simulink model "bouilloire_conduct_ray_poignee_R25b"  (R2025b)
settings: Solver=VariableStepAuto  StartTime=0.0  StopTime=2000  RelTol=1e-3  AbsTol=1e-3  EnableMultiTasking=on
PreLoadFcn:
  | % Caractéristiques de la poignée en polypropylène
  | D= 0.027;         % [m]  Diamètre moyen
  | L1= 0.03;         % [m]  Longueur des tronçons d'extrémité
  | L2= 0.11;         % [m]  Longueur du tronçon central
  | A= pi*D^2/4;      % [m^2] Surface de la section
  | A_cyl1= pi*D*L1;  % [m^2] Surface cylindre des tronçons d'extrémité
  | A_cyl2= pi*D*L2;  % [m^2] Surface cylindre du tronçon central
  | k= 0.2;           % [W/(K*m)] Conductivité thermique
  | m1= 900*A*L1;     % [kg] Masse tronçons d'extrémité (Masse vol = 900 kg/m3)
  | m2= 900*A*L2;     % [kg] Masse tronçon central
  | c= 1700;          % [J/kg/K] Chaleur spécifique
  | h= 6.8;           % [W/(m^2/K)] Coefficient de convection thermique
  | T_air= 20;        % [degC]
  | T_base= 80;       % [degC]
  | T_init= 20;       % [degC]
  | % Point de fusion du polypropylène = 160 degC
  | e= 0.94;          % Emissivité du plastique noir
libraries: fl_lib x31, nesl_utility x7

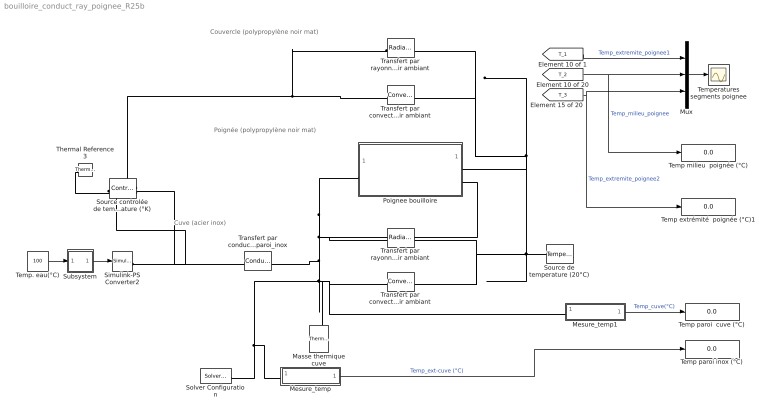
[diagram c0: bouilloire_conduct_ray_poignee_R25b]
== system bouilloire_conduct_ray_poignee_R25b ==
  note: Poignée (polypropylène noir mat)
  note: Cuve (acier inox)
  note: Couvercle (polypropylène noir mat)
  Masse thermique cuve : fl_lib/Thermal/Thermal Elements/Thermal Mass  mass_type=foundation.enum.constant_variable.constant  mass=0.17 kg  sp_heat=470 J/kg/K  mass_min=1e-6 kg  num_ports=foundation.enum.numPorts2.one  m_specify=off  m_priority=High  m=1 kg  m_nominal_specify=off  m_nominal_value=1  m_nominal_unit=kg  T_specify=on  T_priority=High  T=293 K  T_nominal_specify=off  T_nominal_value=1  T_nominal_unit=K  Q_specify=on  Q_priority=None  Q=0 W  Q_nominal_specify=off  Q_nominal_value=1  Q_nominal_unit=W
  Mesure_temp : Subsystem
  Mesure_temp1 : Subsystem
  Mux : Mux  Inputs=3
  Poignee bouilloire : Subsystem  Tag=PublishSubsystem
  Simulink-PS Converter2 : nesl_utility/Simulink-PS Converter  PhysicalDomain=network_engine_domain  SubClassName=ps_input  LeftPortType=input  RightPortType=output  PseudoPeriodic=off  Frequencies=[]  NoiseDistribution=none  NoiseParameters=[]  Unit=1  AffineConversion=off  FilteringAndDerivatives=zero  SimscapeFilterOrder=1  InputFilterTimeConstant=0.001  UdotUserProvided=1
  Solver Configuration : nesl_utility/Solver Configuration  PhysicalDomain=network_engine_domain  SubClassName=solver  LeftPortType=input  RightPortType=generic  Tones=[]  Harmonics=[]  SimulateNoise=off  Profile=off  UseLocalSampling=off  EnableSwitchedLinearOptims=on  FrequencyDomain=off  UseCCode=off  RelTol=0.001  AbsTol=1e-06  MinStep=1e-09  ToWorkspace=off  RevertToSquareIcSolve=off  NumHomotopyIterations=100  PhasorMode=off  PhasorModeNumHarmonics=1  ConsistencySolver=NEWTON_FTOL  IndexReductionMethod=DerivativeReplacement  DoDC=off  ResidualTolerance=1e-09  ConsistencyTolSource=GLOBAL  ConsistencyAbsTol=0.001  ConsistencyRelTol=0.001  ConsistencyTolFactor=0.001  UseLocalSolver=off  LocalSolverChoice=NE_BACKWARD_EULER_ADVANCER  ResolveIndetEquations=on  FunctionEvalNumThread=1  LocalSolverSampleTime=0.001  DoFixedCost=off  MaxNonlinIter=3  MaxModeIter=2  ComputeImpulses=off  ImpulseIterations=2  LinearAlgebra=Sparse  LinearAlgebraNumThread=0  EquationFormulation=NE_TIME_EF  DelaysMemoryBudget=1024  AutomaticFiltering=on  FilteringTimeConstant=0.001  PartitionStorageMethod=AS_NEEDED  PartitionMemoryBudget=1024  PartitionMethod=FAST  MultibodyUseLocalSolver=off  MultibodyLocalSolverChoice=ODE1  MultibodyLocalSolverSampleTime=0.001
  Source controlée de temperature (°K) : fl_lib/Thermal/Thermal Sources/Controlled Temperature Source
  Source de temperature (20°C) : fl_lib/Thermal/Thermal Sources/Temperature Source  temperature=293.15 K
  Subsystem : Subsystem
  Temp extrémité  poignée (°C)1 : Display
  Temp milieu  poignée (°C) : Display
  Temp paroi  cuve (°C) : Display
  Temp paroi inox (°C) : Display
  Temp. eau(°C) : Constant  Value=100
  Temperatures segments poignee : Scope
  Thermal Reference3 : fl_lib/Thermal/Thermal Elements/Thermal Reference
  Transfert par conduction eau-paroi_inox : fl_lib/Thermal/Thermal Elements/Conductive Heat Transfer  thermal_type=foundation.enum.ConstantVariableTabulated.Constant  wall_geometry=foundation.enum.ConductionWallGeometry.Planar  area=53e-3 m^2  thickness=0.4 mm  d_in=0.05 m  d_out=0.1 m  L=1 m  th_cond_min=10 W/(K*m)  th_cond=17 W/(m*K)  th_cond_TLU=[413, 401, 392, 383, 371, 357, 342] W/(K*m)  temp_TLU=[200, 273, 400, 600, 800, 1000, 1200] K  T_specify=off  T_priority=None  T=0 K  T_nominal_specify=off  T_nominal_value=1  T_nominal_unit=K  Q_specify=off  Q_priority=None  Q=0 W  Q_nominal_specify=off  Q_nominal_value=1  Q_nominal_unit=W
  Transfert par convection couvercle-air ambiant : fl_lib/Thermal/Thermal Elements/Convective Heat Transfer  thermal_type=foundation.enum.constant_variable.constant  area=8e-3 m^2  heat_tr_coeff=6.8 W/(m^2 * K)  min_heat_tr_coeff=1e-3 W/(K*m^2)  T_specify=off  T_priority=None  T=0 K  T_nominal_specify=off  T_nominal_value=1  T_nominal_unit=K  Q_specify=off  Q_priority=None  Q=0 W  Q_nominal_specify=off  Q_nominal_value=1  Q_nominal_unit=W
  Transfert par convection paroi_inox-air ambiant : fl_lib/Thermal/Thermal Elements/Convective Heat Transfer  thermal_type=foundation.enum.constant_variable.constant  area=53e-3 m^2  heat_tr_coeff=6.8 W/(m^2 * K)  min_heat_tr_coeff=1e-3 W/(K*m^2)  T_specify=off  T_priority=None  T=0 K  T_nominal_specify=off  T_nominal_value=1  T_nominal_unit=K  Q_specify=off  Q_priority=None  Q=0 W  Q_nominal_specify=off  Q_nominal_value=1  Q_nominal_unit=W
  Transfert par rayonnement couvercle-air ambiant : fl_lib/Thermal/Thermal Elements/Radiative Heat Transfer  area=8e-3 m^2  rad_tr_coeff=e*5.67e-8 W/(m^2*K^4)  T_specify=off  T_priority=None  T=0 K  T_nominal_specify=off  T_nominal_value=1  T_nominal_unit=K  Q_specify=off  Q_priority=None  Q=0 W  Q_nominal_specify=off  Q_nominal_value=1  Q_nominal_unit=W
  Transfert par rayonnement paroi_inox-air ambiant : fl_lib/Thermal/Thermal Elements/Radiative Heat Transfer  area=53e-3 m^2  rad_tr_coeff=0.87*5.67e-8 W/(m^2*K^4)  T_specify=off  T_priority=None  T=0 K  T_nominal_specify=off  T_nominal_value=1  T_nominal_unit=K  Q_specify=off  Q_priority=None  Q=0 W  Q_nominal_specify=off  Q_nominal_value=1  Q_nominal_unit=W
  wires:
  Mesure_temp/1(Temp(°C)) -> Temp paroi inox (°C)/1  "Temp_ext-cuve (°C)"
  Mesure_temp1/1(Temp(°C)) -> Temp paroi  cuve (°C)/1  "Temp_cuve(°C)"
  Subsystem/1(S1) -> Simulink-PS Converter2/1
  Temp. eau(°C)/1 -> Subsystem/1(E1)
  [T_2] -> Mux/2, Temp milieu  poignée (°C)/1  "Temp_milieu_poignee"
  [T_3] -> Mux/3, Temp extrémité  poignée (°C)1/1  "Temp_extremite_poignee2"
  [T_1] -> Mux/1  "Temp_extremite_poignee1"
  Mux/1 -> Temperatures segments poignee/1
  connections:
  Poignee bouilloire/LConn1 -- Poignee bouilloire/RConn2 -- Transfert par rayonnement paroi_inox-air ambiant/LConn1 -- Transfert par conduction eau-paroi_inox/RConn1 -- Mesure_temp/LConn1 -- Solver Configuration/RConn1 -- Mesure_temp1/LConn1 -- Masse thermique cuve/LConn1 -- Transfert par convection paroi_inox-air ambiant/LConn1
  Transfert par convection couvercle-air ambiant/RConn1 -- Transfert par rayonnement couvercle-air ambiant/RConn1 -- Source de temperature (20°C)/LConn1 -- Transfert par convection paroi_inox-air ambiant/RConn1 -- Transfert par rayonnement paroi_inox-air ambiant/RConn1 -- Poignee bouilloire/RConn1
  Thermal Reference3/LConn1 -- Source controlée de temperature (°K)/RConn2
  Source controlée de temperature (°K)/RConn1 -- Simulink-PS Converter2/RConn1
  Source controlée de temperature (°K)/LConn1 -- Transfert par conduction eau-paroi_inox/LConn1 -- Transfert par convection couvercle-air ambiant/LConn1 -- Transfert par rayonnement couvercle-air ambiant/LConn1

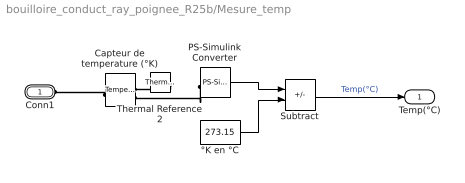
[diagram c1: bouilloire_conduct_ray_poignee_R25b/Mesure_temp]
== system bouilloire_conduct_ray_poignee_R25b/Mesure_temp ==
  Capteur de temperature (°K) : fl_lib/Thermal/Thermal Sensors/Temperature Sensor  temperature_measure=foundation.enum.MeasurementReference.difference
  PS-Simulink Converter : nesl_utility/PS-Simulink Converter  PhysicalDomain=network_engine_domain  SubClassName=ps_output  LeftPortType=input  RightPortType=output  PseudoPeriodic=off  Frequencies=[]  VectorFormat=1-D array  Unit=1  AffineConversion=off
  Subtract : Sum  Inputs=+-
  Thermal Reference2 : fl_lib/Thermal/Thermal Elements/Thermal Reference
  °K en °C : Constant  Value=273.15
  Conn1 : PMIOPort  Side=Left
  Temp(°C) : Outport  VectorParamsAs1DForOutWhenUnconnected=off
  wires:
  °K en °C/1 -> Subtract/2
  Subtract/1 -> Temp(°C)/1  "Temp(°C)"
  PS-Simulink Converter/1 -> Subtract/1
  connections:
  PS-Simulink Converter/LConn1 -- Capteur de temperature (°K)/RConn2
  Thermal Reference2/LConn1 -- Capteur de temperature (°K)/RConn1
  Capteur de temperature (°K)/LConn1 -- Conn1/RConn1

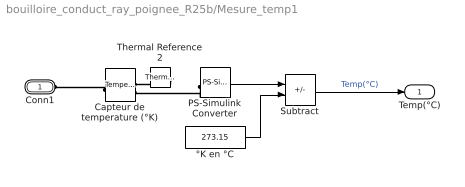
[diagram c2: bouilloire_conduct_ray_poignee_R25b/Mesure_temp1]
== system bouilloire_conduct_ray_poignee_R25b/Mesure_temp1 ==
  Capteur de temperature (°K) : fl_lib/Thermal/Thermal Sensors/Temperature Sensor  temperature_measure=foundation.enum.MeasurementReference.difference
  PS-Simulink Converter : nesl_utility/PS-Simulink Converter  PhysicalDomain=network_engine_domain  SubClassName=ps_output  LeftPortType=input  RightPortType=output  PseudoPeriodic=off  Frequencies=[]  VectorFormat=1-D array  Unit=1  AffineConversion=off
  Subtract : Sum  Inputs=+-
  Thermal Reference2 : fl_lib/Thermal/Thermal Elements/Thermal Reference
  °K en °C : Constant  Value=273.15
  Conn1 : PMIOPort  Side=Left
  Temp(°C) : Outport  VectorParamsAs1DForOutWhenUnconnected=off
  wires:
  °K en °C/1 -> Subtract/2
  Subtract/1 -> Temp(°C)/1  "Temp(°C)"
  PS-Simulink Converter/1 -> Subtract/1
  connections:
  PS-Simulink Converter/LConn1 -- Capteur de temperature (°K)/RConn2
  Thermal Reference2/LConn1 -- Capteur de temperature (°K)/RConn1
  Capteur de temperature (°K)/LConn1 -- Conn1/RConn1

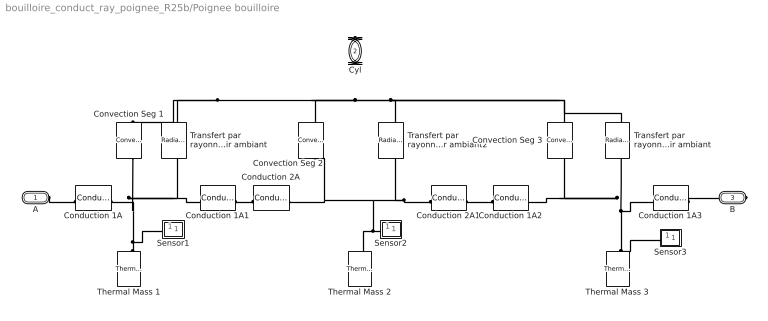
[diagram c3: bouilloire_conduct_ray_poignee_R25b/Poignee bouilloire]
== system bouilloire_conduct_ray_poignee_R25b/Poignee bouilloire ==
  Conduction 1A{,1..3} (4 alike) : fl_lib/Thermal/Thermal Elements/Conductive Heat Transfer  thermal_type=foundation.enum.ConstantVariableTabulated.Constant  wall_geometry=foundation.enum.ConductionWallGeometry.Planar  area=A m^2  thickness=L1/2 m  d_in=0.05 m  d_out=0.1 m  L=1 m  th_cond_min=10 W/(K*m)  th_cond=k W/m/K  th_cond_TLU=[413, 401, 392, 383, 371, 357, 342] W/(K*m)  temp_TLU=[200, 273, 400, 600, 800, 1000, 1200] K  T_specify=off  T_priority=High  T=0 K  T_nominal_specify=off  T_nominal_value=1  T_nominal_unit=K  Q_specify=off  Q_priority=High  Q=0 J/s  Q_nominal_specify=off  Q_nominal_value=1  Q_nominal_unit=J/s
  Conduction 2A : fl_lib/Thermal/Thermal Elements/Conductive Heat Transfer  thermal_type=foundation.enum.ConstantVariableTabulated.Constant  wall_geometry=foundation.enum.ConductionWallGeometry.Planar  area=A m^2  thickness=L2/2 m  d_in=0.05 m  d_out=0.1 m  L=1 m  th_cond_min=10 W/(K*m)  th_cond=k W/m/K  th_cond_TLU=[413, 401, 392, 383, 371, 357, 342] W/(K*m)  temp_TLU=[200, 273, 400, 600, 800, 1000, 1200] K  T_specify=off  T_priority=High  T=0 K  T_nominal_specify=off  T_nominal_value=1  T_nominal_unit=K  Q_specify=off  Q_priority=High  Q=0 J/s  Q_nominal_specify=off  Q_nominal_value=1  Q_nominal_unit=J/s
  Conduction 2A1 : fl_lib/Thermal/Thermal Elements/Conductive Heat Transfer  thermal_type=foundation.enum.ConstantVariableTabulated.Constant  wall_geometry=foundation.enum.ConductionWallGeometry.Planar  area=A m^2  thickness=L2/2 m  d_in=0.05 m  d_out=0.1 m  L=1 m  th_cond_min=10 W/(K*m)  th_cond=k W/m/K  th_cond_TLU=[413, 401, 392, 383, 371, 357, 342] W/(K*m)  temp_TLU=[200, 273, 400, 600, 800, 1000, 1200] K  T_specify=off  T_priority=High  T=0 K  T_nominal_specify=off  T_nominal_value=1  T_nominal_unit=K  Q_specify=off  Q_priority=High  Q=0 J/s  Q_nominal_specify=off  Q_nominal_value=1  Q_nominal_unit=J/s
  Convection Seg 1 : fl_lib/Thermal/Thermal Elements/Convective Heat Transfer  thermal_type=foundation.enum.constant_variable.constant  area=A_cyl1 m^2  heat_tr_coeff=h W/m^2/K  min_heat_tr_coeff=1e-3 W/(K*m^2)  T_specify=off  T_priority=High  T=0 K  T_nominal_specify=off  T_nominal_value=1  T_nominal_unit=K  Q_specify=off  Q_priority=High  Q=0 J/s  Q_nominal_specify=off  Q_nominal_value=1  Q_nominal_unit=J/s
  Convection Seg 2 : fl_lib/Thermal/Thermal Elements/Convective Heat Transfer  thermal_type=foundation.enum.constant_variable.constant  area=A_cyl2 m^2  heat_tr_coeff=h W/m^2/K  min_heat_tr_coeff=1e-3 W/(K*m^2)  T_specify=off  T_priority=High  T=0 K  T_nominal_specify=off  T_nominal_value=1  T_nominal_unit=K  Q_specify=off  Q_priority=High  Q=0 J/s  Q_nominal_specify=off  Q_nominal_value=1  Q_nominal_unit=J/s
  Convection Seg 3 : fl_lib/Thermal/Thermal Elements/Convective Heat Transfer  thermal_type=foundation.enum.constant_variable.constant  area=A_cyl1 m^2  heat_tr_coeff=h W/m^2/K  min_heat_tr_coeff=1e-3 W/(K*m^2)  T_specify=off  T_priority=High  T=0 K  T_nominal_specify=off  T_nominal_value=1  T_nominal_unit=K  Q_specify=off  Q_priority=High  Q=0 J/s  Q_nominal_specify=off  Q_nominal_value=1  Q_nominal_unit=J/s
  Sensor1 : Subsystem
  Sensor2 : Subsystem
  Sensor3 : Subsystem
  Thermal Mass 1 : fl_lib/Thermal/Thermal Elements/Thermal Mass  mass_type=foundation.enum.constant_variable.constant  mass=m1 kg  sp_heat=c J/kg/K  mass_min=1e-6 kg  num_ports=foundation.enum.numPorts2.one  m_specify=off  m_priority=High  m=1 kg  m_nominal_specify=off  m_nominal_value=1  m_nominal_unit=kg  T_specify=on  T_priority=High  T=T_init degC  T_nominal_specify=off  T_nominal_value=1  T_nominal_unit=K  Q_specify=off  Q_priority=None  Q=0 W  Q_nominal_specify=off  Q_nominal_value=1  Q_nominal_unit=W
  Thermal Mass 2 : fl_lib/Thermal/Thermal Elements/Thermal Mass  mass_type=foundation.enum.constant_variable.constant  mass=m2 kg  sp_heat=c J/kg/K  mass_min=1e-6 kg  num_ports=foundation.enum.numPorts2.one  m_specify=off  m_priority=High  m=1 kg  m_nominal_specify=off  m_nominal_value=1  m_nominal_unit=kg  T_specify=on  T_priority=High  T=T_init degC  T_nominal_specify=off  T_nominal_value=1  T_nominal_unit=K  Q_specify=off  Q_priority=None  Q=0 W  Q_nominal_specify=off  Q_nominal_value=1  Q_nominal_unit=W
  Thermal Mass 3 : fl_lib/Thermal/Thermal Elements/Thermal Mass  mass_type=foundation.enum.constant_variable.constant  mass=m1 kg  sp_heat=c J/kg/K  mass_min=1e-6 kg  num_ports=foundation.enum.numPorts2.one  m_specify=off  m_priority=High  m=1 kg  m_nominal_specify=off  m_nominal_value=1  m_nominal_unit=kg  T_specify=on  T_priority=High  T=T_init degC  T_nominal_specify=off  T_nominal_value=1  T_nominal_unit=K  Q_specify=off  Q_priority=None  Q=0 W  Q_nominal_specify=off  Q_nominal_value=1  Q_nominal_unit=W
  Transfert par rayonnement seg1-air ambiant : fl_lib/Thermal/Thermal Elements/Radiative Heat Transfer  area=A_cyl1 m^2  rad_tr_coeff=e*5.67e-8 W/(m^2*K^4)  T_specify=off  T_priority=None  T=0 K  T_nominal_specify=off  T_nominal_value=1  T_nominal_unit=K  Q_specify=off  Q_priority=None  Q=0 W  Q_nominal_specify=off  Q_nominal_value=1  Q_nominal_unit=W
  Transfert par rayonnement seg2-air ambiant2 : fl_lib/Thermal/Thermal Elements/Radiative Heat Transfer  area=A_cyl2 m^2  rad_tr_coeff=e*5.67e-8 W/(m^2*K^4)  T_specify=off  T_priority=None  T=0 K  T_nominal_specify=off  T_nominal_value=1  T_nominal_unit=K  Q_specify=off  Q_priority=None  Q=0 W  Q_nominal_specify=off  Q_nominal_value=1  Q_nominal_unit=W
  Transfert par rayonnement seg3-air ambiant : fl_lib/Thermal/Thermal Elements/Radiative Heat Transfer  area=A_cyl1 m^2  rad_tr_coeff=e*5.67e-8 W/(m^2*K^4)  T_specify=off  T_priority=None  T=0 K  T_nominal_specify=off  T_nominal_value=1  T_nominal_unit=K  Q_specify=off  Q_priority=None  Q=0 W  Q_nominal_specify=off  Q_nominal_value=1  Q_nominal_unit=W
  A : PMIOPort  Side=Left
  Cyl : PMIOPort  Port=2  Side=Right
  B : PMIOPort  Port=3  Side=Right
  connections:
  Conduction 2A1/RConn1 -- Conduction 1A2/LConn1
  A/RConn1 -- Conduction 1A/LConn1
  Conduction 2A/LConn1 -- Conduction 1A1/RConn1
  Thermal Mass 3/LConn1 -- Transfert par rayonnement seg3-air ambiant/LConn1 -- Convection Seg 3/LConn1 -- Conduction 1A2/RConn1 -- Conduction 1A3/LConn1 -- Sensor3/LConn1
  Sensor2/LConn1 -- Thermal Mass 2/LConn1 -- Conduction 2A/RConn1 -- Convection Seg 2/LConn1 -- Conduction 2A1/LConn1 -- Transfert par rayonnement seg2-air ambiant2/LConn1
  Thermal Mass 1/LConn1 -- Sensor1/LConn1 -- Transfert par rayonnement seg1-air ambiant/LConn1 -- Conduction 1A1/LConn1 -- Conduction 1A/RConn1 -- Convection Seg 1/LConn1
  Conduction 1A3/RConn1 -- B/RConn1
  Cyl/RConn1 -- Convection Seg 2/RConn1 -- Transfert par rayonnement seg1-air ambiant/RConn1 -- Convection Seg 1/RConn1 -- Transfert par rayonnement seg3-air ambiant/RConn1 -- Convection Seg 3/RConn1 -- Transfert par rayonnement seg2-air ambiant2/RConn1

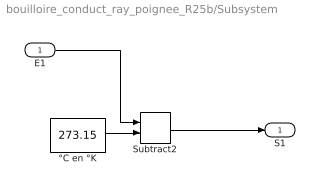
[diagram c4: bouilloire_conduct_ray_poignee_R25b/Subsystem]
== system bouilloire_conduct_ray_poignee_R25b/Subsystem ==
  E1 : Inport
  Subtract2 : Sum
  °C en °K : Constant  Value=273.15
  S1 : Outport  VectorParamsAs1DForOutWhenUnconnected=off
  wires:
  °C en °K/1 -> Subtract2/2
  Subtract2/1 -> S1/1
  E1/1 -> Subtract2/1

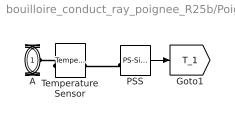
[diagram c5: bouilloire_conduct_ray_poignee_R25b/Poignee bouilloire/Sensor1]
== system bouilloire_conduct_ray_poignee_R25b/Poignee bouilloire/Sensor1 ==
  PSS : nesl_utility/PS-Simulink Converter  PhysicalDomain=network_engine_domain  SubClassName=ps_output  LeftPortType=input  RightPortType=output  PseudoPeriodic=off  Frequencies=[]  VectorFormat=1-D array  Unit=degC  AffineConversion=on
  Temperature Sensor : fl_lib/Thermal/Thermal Sensors/Temperature Sensor  temperature_measure=foundation.enum.MeasurementReference.absolute
  A : PMIOPort  Side=Left
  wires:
  PSS/1 -> [T_1]
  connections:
  PSS/LConn1 -- Temperature Sensor/RConn1
  Temperature Sensor/LConn1 -- A/RConn1

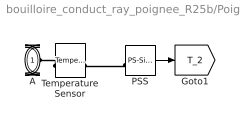
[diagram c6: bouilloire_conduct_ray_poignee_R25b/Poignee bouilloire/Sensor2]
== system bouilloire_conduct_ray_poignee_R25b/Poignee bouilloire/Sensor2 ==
  PSS : nesl_utility/PS-Simulink Converter  PhysicalDomain=network_engine_domain  SubClassName=ps_output  LeftPortType=input  RightPortType=output  PseudoPeriodic=off  Frequencies=[]  VectorFormat=1-D array  Unit=degC  AffineConversion=on
  Temperature Sensor : fl_lib/Thermal/Thermal Sensors/Temperature Sensor  temperature_measure=foundation.enum.MeasurementReference.absolute
  A : PMIOPort  Side=Left
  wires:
  PSS/1 -> [T_2]
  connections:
  PSS/LConn1 -- Temperature Sensor/RConn1
  Temperature Sensor/LConn1 -- A/RConn1

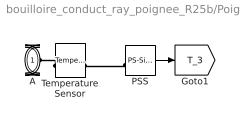
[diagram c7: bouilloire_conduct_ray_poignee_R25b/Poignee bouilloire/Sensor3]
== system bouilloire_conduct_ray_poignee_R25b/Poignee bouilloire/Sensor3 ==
  PSS : nesl_utility/PS-Simulink Converter  PhysicalDomain=network_engine_domain  SubClassName=ps_output  LeftPortType=input  RightPortType=output  PseudoPeriodic=off  Frequencies=[]  VectorFormat=1-D array  Unit=degC  AffineConversion=on
  Temperature Sensor : fl_lib/Thermal/Thermal Sensors/Temperature Sensor  temperature_measure=foundation.enum.MeasurementReference.absolute
  A : PMIOPort  Side=Left
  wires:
  PSS/1 -> [T_3]
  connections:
  PSS/LConn1 -- Temperature Sensor/RConn1
  Temperature Sensor/LConn1 -- A/RConn1
